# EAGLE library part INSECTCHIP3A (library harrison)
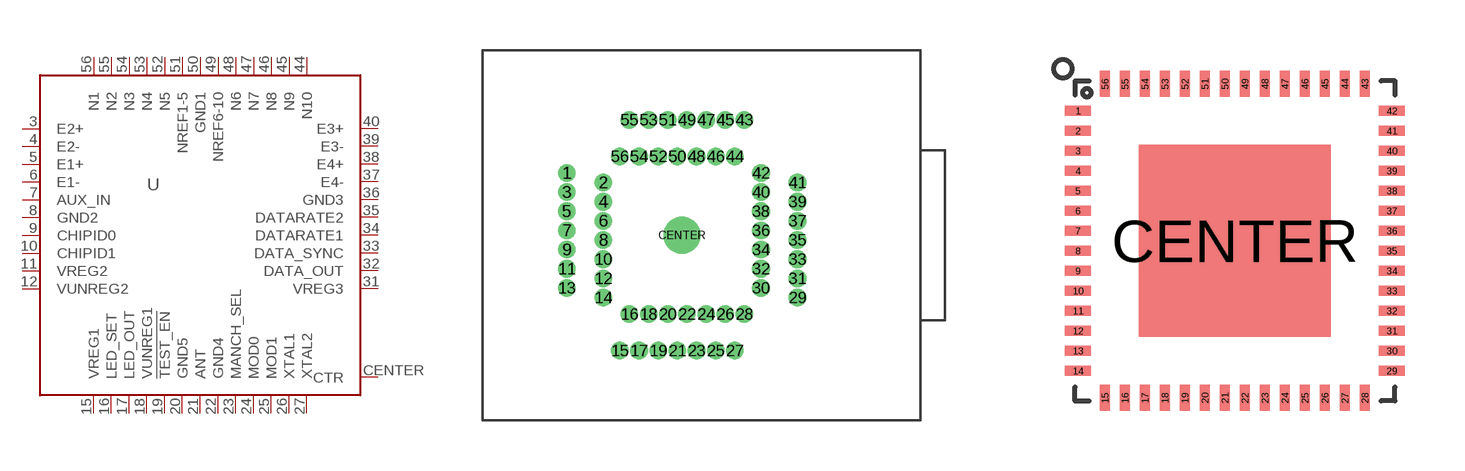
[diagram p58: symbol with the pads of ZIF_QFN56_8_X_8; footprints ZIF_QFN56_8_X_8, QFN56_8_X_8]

Designator prefix U

## INSECTCHIP3A_ZIF  [ZIF_QFN56_8_X_8]
3  E2+  in
4  E2-  in
5  E1+  in
6  E1-  in
7  AUX_IN  in
8  GND2  pwr
9  CHIPID0  in
10  CHIPID1  in
11  VREG2  pwr
12  VUNREG2  pwr
15  VREG1  pwr
16  LED_SET  pas
17  LED_OUT  pas
18  VUNREG1  pwr
19  !TEST_EN!  in
20  GND5  pwr
21  ANT  pas
22  GND4  pwr
23  MANCH_SEL  in
24  MOD0  in
25  MOD1  in
26  XTAL1  pas
27  XTAL2  pas
31  VREG3  pwr
32  DATA_OUT  out
33  DATA_SYNC  out
34  DATARATE1  in
35  DATARATE2  in
36  GND3  pwr
37  E4-  in
38  E4+  in
39  E3-  in
40  E3+  in
44  N10  in
45  N9  in
46  N8  in
47  N7  in
48  N6  in
49  NREF6-10  in
50  GND1  pwr
51  NREF1-5  in
52  N5  in
53  N4  in
54  N3  in
55  N2  in
56  N1  in
CENTER  CTR  pwr

## INSECTCHIP3A_QFN  [QFN56_8_X_8]
Pads as for ZIF_QFN56_8_X_8

## INSECTCHIP3A_COB1  [INSECTCHIP3_COB_1]
1  E2+  in
2  E2-  in
3  E1+  in
4  E1-  in
5  AUX_IN  in
6  GND2  pwr
7  CHIPID0  in
8  CHIPID1  in
9  VREG2  pwr
10  VUNREG2  pwr
11  VREG1  pwr
12  LED_SET  pas
13  LED_OUT  pas
14  VUNREG1  pwr
15  !TEST_EN!  in
16  GND5  pwr
17  ANT  pas
18  GND4  pwr
19  MANCH_SEL  in
20  MOD0  in
21  MOD1  in
22  XTAL1  pas
23  XTAL2  pas
24  VREG3  pwr
25  DATA_OUT  out
26  DATA_SYNC  out
27  DATARATE1  in
28  DATARATE2  in
29  GND3  pwr
30  E4-  in
31  E4+  in
32  E3-  in
33  E3+  in
34  N10  in
35  N9  in
36  N8  in
37  N7  in
38  N6  in
39  NREF6-10  in
40  GND1  pwr
41  NREF1-5  in
42  N5  in
43  N4  in
44  N3  in
45  N2  in
46  N1  in
CENTER  CTR  pwr

## INSECTCHIP3A_COB2  [INSECTCHIP3_COB_2]
Pads as for INSECTCHIP3_COB_1

## Footprint ZIF_QFN56_8_X_8 (pad centres in mm)
drill 0.41 pad 0.813: 1 -6.02,3.251; 2 -4.115,2.751; 3 -6.02,2.25; 4 -4.115,1.75; 5 -6.02,1.25; 6 -4.115,0.752; 7 -6.02,0.249; 8 -4.115,-0.249; 9 -6.02,-0.749; 10 -4.115,-1.25; 11 -6.02,-1.75; 12 -4.115,-2.25; 13 -6.02,-2.751; 14 -4.115,-3.251; 15 -3.251,-6.02; 16 -2.751,-4.115; 17 -2.25,-6.02; 18 -1.75,-4.115; 19 -1.25,-6.02; 20 -0.752,-4.115; 21 -0.249,-6.02; 22 0.249,-4.115; 23 0.749,-6.02; 24 1.25,-4.115; 25 1.75,-6.02; 26 2.25,-4.115; 27 2.751,-6.02; 28 3.251,-4.115; 29 6.02,-3.251; 30 4.115,-2.751; 31 6.02,-2.25; 32 4.115,-1.75; 33 6.02,-1.25; 34 4.115,-0.752; 35 6.02,-0.249; 36 4.115,0.249; 37 6.02,0.749; 38 4.115,1.25; 39 6.02,1.75; 40 4.115,2.25; 41 6.02,2.751; 42 4.115,3.251; 43 3.251,6.02; 44 2.751,4.115; 45 2.25,6.02; 46 1.75,4.115; 47 1.25,6.02; 48 0.752,4.115; 49 0.249,6.02; 50 -0.249,4.115; 51 -0.749,6.02; 52 -1.25,4.115; 53 -1.75,6.02; 54 -2.25,4.115; 55 -2.751,6.02; 56 -3.251,4.115
drill 1.02 pad 1.93: CENTER 0,0

## Footprint QFN56_8_X_8 (pad centres in mm)
smd 0.65 x 0.25: 1 -3.925,3.25; 2 -3.925,2.75; 3 -3.925,2.25; 4 -3.925,1.75; 5 -3.925,1.25; 6 -3.925,0.75; 7 -3.925,0.25; 8 -3.925,-0.25; 9 -3.925,-0.75; 10 -3.925,-1.25; 11 -3.925,-1.75; 12 -3.925,-2.25; 13 -3.925,-2.75; 14 -3.925,-3.25; 29 3.925,-3.25; 30 3.925,-2.75; 31 3.925,-2.25; 32 3.925,-1.75; 33 3.925,-1.25; 34 3.925,-0.75; 35 3.925,-0.25; 36 3.925,0.25; 37 3.925,0.75; 38 3.925,1.25; 39 3.925,1.75; 40 3.925,2.25; 41 3.925,2.75; 42 3.925,3.25
smd 0.25 x 0.65: 15 -3.25,-3.925; 16 -2.75,-3.925; 17 -2.25,-3.925; 18 -1.75,-3.925; 19 -1.25,-3.925; 20 -0.75,-3.925; 21 -0.25,-3.925; 22 0.25,-3.925; 23 0.75,-3.925; 24 1.25,-3.925; 25 1.75,-3.925; 26 2.25,-3.925; 27 2.75,-3.925; 28 3.25,-3.925; 43 3.25,3.925; 44 2.75,3.925; 45 2.25,3.925; 46 1.75,3.925; 47 1.25,3.925; 48 0.75,3.925; 49 0.25,3.925; 50 -0.25,3.925; 51 -0.75,3.925; 52 -1.25,3.925; 53 -1.75,3.925; 54 -2.25,3.925; 55 -2.75,3.925; 56 -3.25,3.925
smd 4.8 x 4.8: CENTER 0,0

## Footprint INSECTCHIP3_COB_1 (pad centres in mm)
smd 0.254 x 0.152: 1 -1.968,1.143; 2 -1.968,0.889; 3 -1.968,0.635; 4 -1.968,0.381; 5 -1.968,0.127; 6 -1.968,-0.127; 7 -1.968,-0.381; 8 -1.968,-0.635; 9 -1.968,-0.889; 10 -1.968,-1.143; 24 1.968,-1.143; 25 1.968,-0.889; 26 1.968,-0.635; 27 1.968,-0.381; 28 1.968,-0.127; 29 1.968,0.127; 30 1.968,0.381; 31 1.968,0.635; 32 1.968,0.889; 33 1.968,1.143
smd 0.152 x 0.254: 11 -1.524,-1.714; 12 -1.27,-1.714; 13 -1.016,-1.714; 14 -0.762,-1.714; 15 -0.508,-1.714; 16 -0.254,-1.714; 17 0,-1.714; 18 0.254,-1.714; 19 0.508,-1.714; 20 0.762,-1.714; 21 1.016,-1.714; 22 1.27,-1.714; 23 1.524,-1.714; 34 1.524,1.714; 35 1.27,1.714; 36 1.016,1.714; 37 0.762,1.714; 38 0.508,1.714; 39 0.254,1.714; 40 0,1.714; 41 -0.254,1.714; 42 -0.508,1.714; 43 -0.762,1.714; 44 -1.016,1.714; 45 -1.27,1.714; 46 -1.524,1.714
smd 2.921 x 2.413: CENTER 0,0

## Footprint INSECTCHIP3_COB_2 (pad centres in mm)
smd 0.152 x 0.152: 1 -1.778,1.143; 2 -1.778,0.889; 3 -1.778,0.635; 4 -1.778,0.381; 5 -1.778,0.127; 6 -1.778,-0.127; 7 -1.778,-0.381; 8 -1.778,-0.635; 9 -1.778,-0.889; 10 -1.778,-1.143; 11 -1.524,-1.524; 12 -1.27,-1.524; 13 -1.016,-1.524; 14 -0.762,-1.524; 15 -0.508,-1.524; 16 -0.254,-1.524; 17 0,-1.524; 18 0.254,-1.524; 19 0.508,-1.524; 20 0.762,-1.524; 21 1.016,-1.524; 22 1.27,-1.524; 23 1.524,-1.524; 24 1.778,-1.143; 25 1.778,-0.889; 26 1.778,-0.635; 27 1.778,-0.381; 28 1.778,-0.127; 29 1.778,0.127; 30 1.778,0.381; 31 1.778,0.635; 32 1.778,0.889; 33 1.778,1.143; 34 1.524,1.524; 35 1.27,1.524; 36 1.016,1.524; 37 0.762,1.524; 38 0.508,1.524; 39 0.254,1.524; 40 0,1.524; 41 -0.254,1.524; 42 -0.508,1.524; 43 -0.762,1.524; 44 -1.016,1.524; 45 -1.27,1.524; 46 -1.524,1.524
smd 2.54 x 2.032: CENTER 0,0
